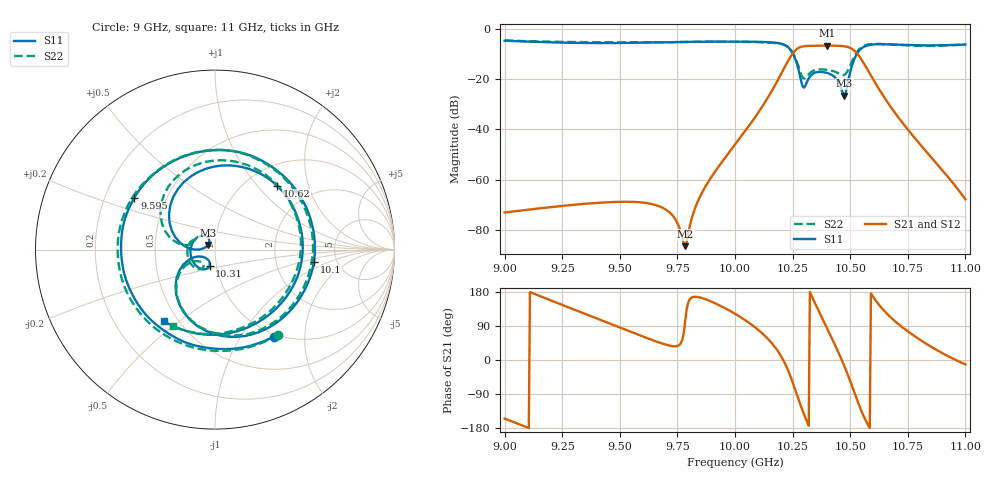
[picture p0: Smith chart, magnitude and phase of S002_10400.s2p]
# Hz S DB R 50
! Planar, S50180, , 20.4.1/1
! Date: 14.11.2021 11:30:39
! Data: Format (Calibration Info)
! Freq	S11:dB/Ang(--)	S21:dB/Ang(--)	S12:dB/Ang(--)	S22:dB/Ang(--)
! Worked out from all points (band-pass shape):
!   401 points, 9 GHz to 11 GHz, reference 50 ohm
!   highest |S21| = -6.61 dB at 10.4 GHz (marker M1); lowest = -86.5 dB at 9.785 GHz (marker M2)
!   |S21| within 3 dB of the highest: 10.25 GHz to 10.53 GHz (277 MHz wide, 2.67 % of centre)
!   lowest |S11| = -26.5 dB at 10.47 GHz (marker M3), VSWR 1.10, Z = 46.1 + j2.34 ohm
!   |S11| at or under -10 dB: 10.25 GHz to 10.53 GHz (276.5 MHz wide, 2.66 % of centre)
!   |S22| runs from -19.7 to -4.6 dB; largest |S21 - S12| = 0.00047
!   S11 on the Smith chart (normalised r, x): 9 GHz: 0.95, -1.41; 9.595 GHz: 0.33, +0.26; 10.1 GHz: 3.35, -0.65; 10.31 GHz: 0.93, -0.17; 10.62 GHz: 1.36, +1.28; 11 GHz: 0.42, -0.44
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9e9  -4.66 -56.1  -73.10 -154.6  -73.10 -154.6  -4.58 -53.4
9.335e9  -5.57 -143.6  -69.71 125.1  -69.72 125.0  -5.23 -138.1
9.595e9  -5.45 147.2  -69.07 63.2  -69.07 63.1  -5.29 156.2
9.67e9  -5.33 127.6  -70.57 46.4  -70.57 46.3  -5.29 137.6
9.785e9  -5.17 96.8  -86.49 109.1  -86.50 109.1  -5.19 108.0
9.87e9  -5.04 73.1  -63.01 160.8  -63.01 160.7  -5.07 84.2
1e10  -5.02 32.6  -46.06 122.0  -46.07 122.0  -5.14 42.1
1.01e10  -5.12 -7.0  -33.44 79.9  -33.44 79.9  -5.26 -0.3
1.0195e10  -5.76 -66.7  -18.80 15.0  -18.81 15.0  -5.85 -63.7
1.024e10  -8.20 -116.8  -11.18 -41.8  -11.19 -41.8  -8.05 -114.4
1.0275e10  -15.98 -158.6  -7.60 -102.7  -7.60 -102.8  -14.80 -151.9
1.0295e10  -23.12 -138.8  -6.94 -136.4  -6.95 -136.4  -19.50 -140.0
1.0315e10  -20.59 -108.4  -6.76 -166.5  -6.76 -166.6  -18.55 -123.5
1.0335e10  -18.06 -118.9  -6.70 166.0  -6.71 165.9  -16.88 -130.6
1.04e10  -17.53 170.2  -6.61 83.1  -6.62 83.0  -16.29 -179.2
1.0475e10  -26.52 147.5  -6.91 -16.7  -6.92 -16.7  -18.25 161.4
1.0535e10  -9.12 135.5  -10.33 -113.9  -10.34 -113.9  -8.47 143.7
1.0575e10  -6.56 85.6  -16.17 -168.5  -16.18 -168.6  -6.25 100.1
1.062e10  -6.08 45.8  -23.19 149.4  -23.20 149.4  -5.95 61.9
1.067e10  -6.16 13.0  -30.24 115.9  -30.25 115.9  -6.16 28.8
1.083e10  -6.55 -62.9  -48.81 42.9  -48.82 42.9  -6.75 -52.1
1.1e10  -6.20 -125.7  -67.82 -11.7  -67.83 -11.7  -6.23 -119.0
